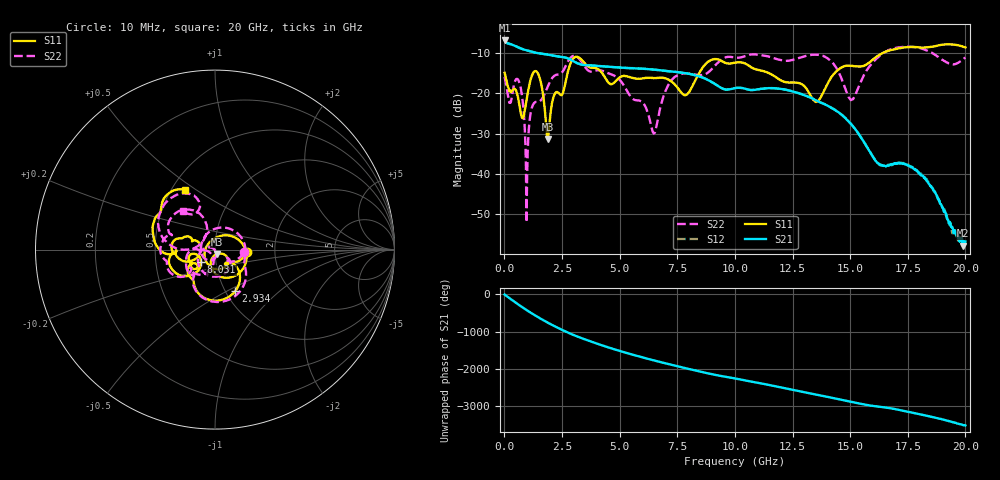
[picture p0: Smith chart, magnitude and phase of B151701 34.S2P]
!  2-Port S-parameters saved by WinCal
! VAR MeasName=S-Parameters (CALIBRATED_DATA) read from VNA (N5244A)
! VAR MeasDate=2015-12-24 19:13:20
! VAR NAME=B151701 34
! VAR FILENAME=B151701 34.S2P
! VAR DATE=2015-12-24 19:13:20
! VAR PHYS_PORTS=1,3
# Hz S DB R 50
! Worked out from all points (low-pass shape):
!   801 points, 10 MHz to 20 GHz, reference 50 ohm
!   highest |S21| = -6.88 dB at 10 MHz (marker M1); lowest = -57.8 dB at 19.88 GHz (marker M2)
!   |S21| within 3 dB of the highest: start of sweep to 1.322 GHz
!   lowest |S11| = -31.3 dB at 1.884 GHz (marker M3), VSWR 1.06, Z = 51.2 - j2.49 ohm
!   |S11| at or under -10 dB: start of sweep to 16.41 GHz
!   |S22| runs from -52.0 to -8.4 dB; largest |S21 - S12| = 0.0014
!   S11 on the Smith chart (normalised r, x): 10 MHz: 1.44, -0.05; 2.934 GHz: 1.11, -0.55; 8.031 GHz: 0.85, -0.12; 20 GHz: 0.59, +0.45
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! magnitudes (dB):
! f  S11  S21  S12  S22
! 10 MHz  -14.9  -6.9  -6.9  -15.9
! 234.9 MHz  -19.2  -7.8  -7.8  -22.1
! 659.7 MHz  -23.2  -8.7  -8.7  -17.5
! 984.5 MHz  -20.8  -9.4  -9.3  -41.4
! 1.184 GHz  -15.7  -9.7  -9.7  -23.7
! 1.434 GHz  -14.9  -10.0  -10.0  -22.1
! 1.884 GHz  -31.3  -10.4  -10.4  -18.3
! 2.934 GHz  -11.8  -11.8  -11.8  -10.8
! 3.358 GHz  -11.7  -12.9  -12.9  -12.3
! 4.958 GHz  -16.2  -13.6  -13.6  -16.4
! 6.457 GHz  -16.2  -14.1  -14.1  -29.8
! 6.682 GHz  -16.2  -14.2  -14.2  -25.7
! 7.206 GHz  -16.9  -14.6  -14.6  -17.1
! 8.031 GHz  -19.5  -15.2  -15.2  -15.1
! 8.881 GHz  -12.0  -16.8  -16.8  -14.6
! 10.01 GHz  -12.4  -18.7  -18.7  -11.1
! 13.35 GHz  -21.2  -21.2  -21.3  -10.4
! 15.05 GHz  -13.2  -27.7  -27.7  -21.6
! 16.68 GHz  -9.4  -37.9  -37.8  -9.3
! 18.2 GHz  -8.7  -40.9  -40.9  -9.1
! 19.88 GHz  -8.4  -57.8  -56.8  -11.7
! 20 GHz  -8.6  -56.7  -57.4  -11.1
